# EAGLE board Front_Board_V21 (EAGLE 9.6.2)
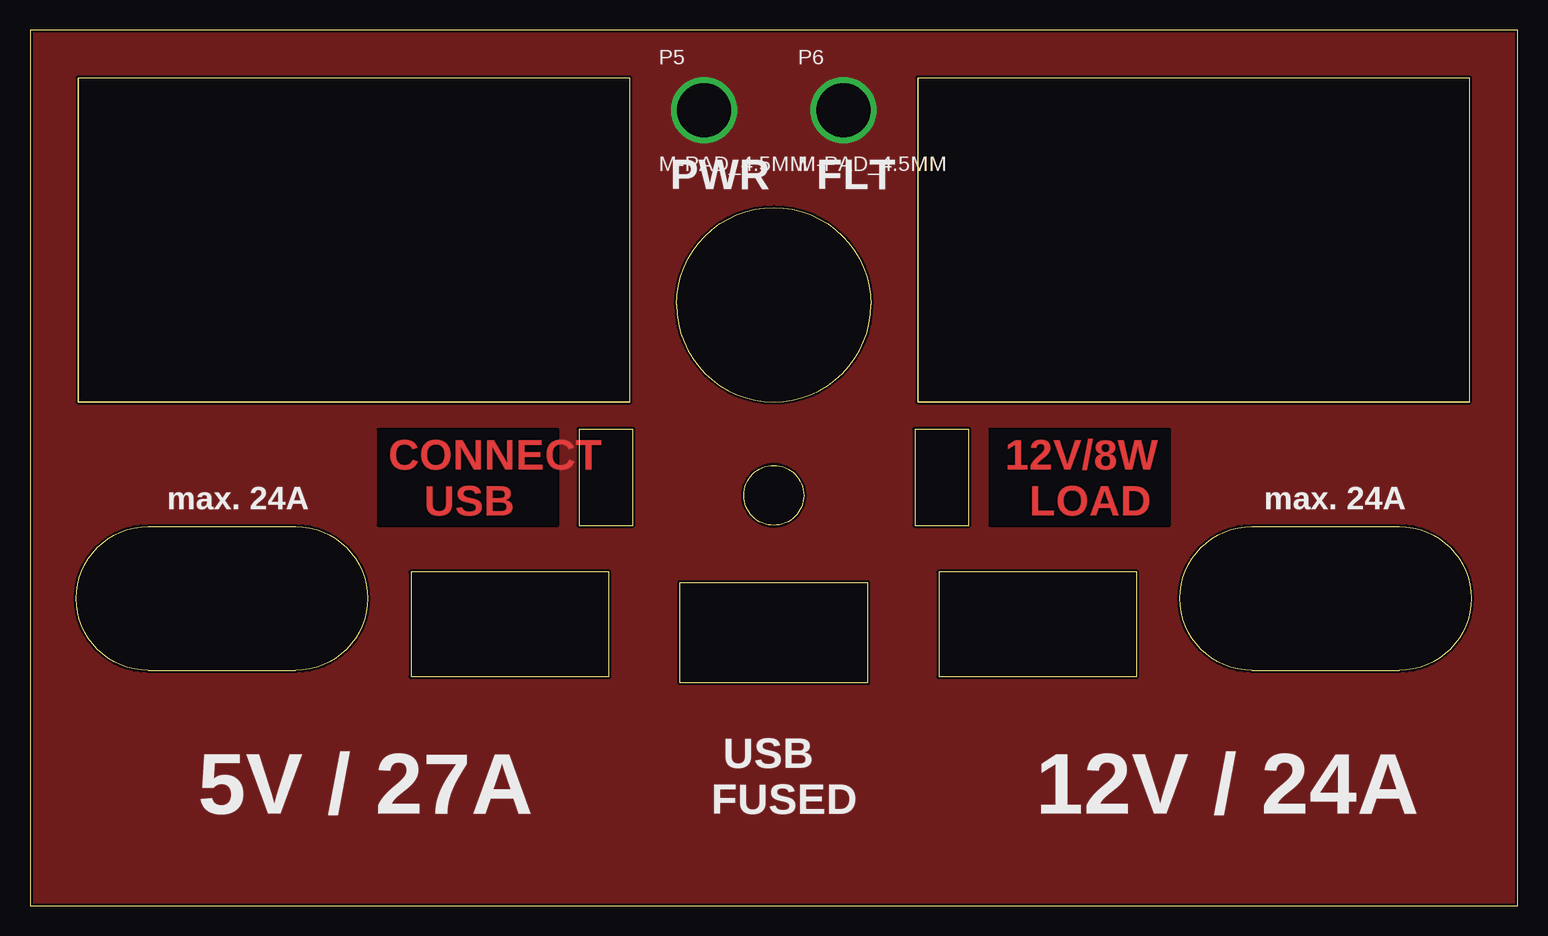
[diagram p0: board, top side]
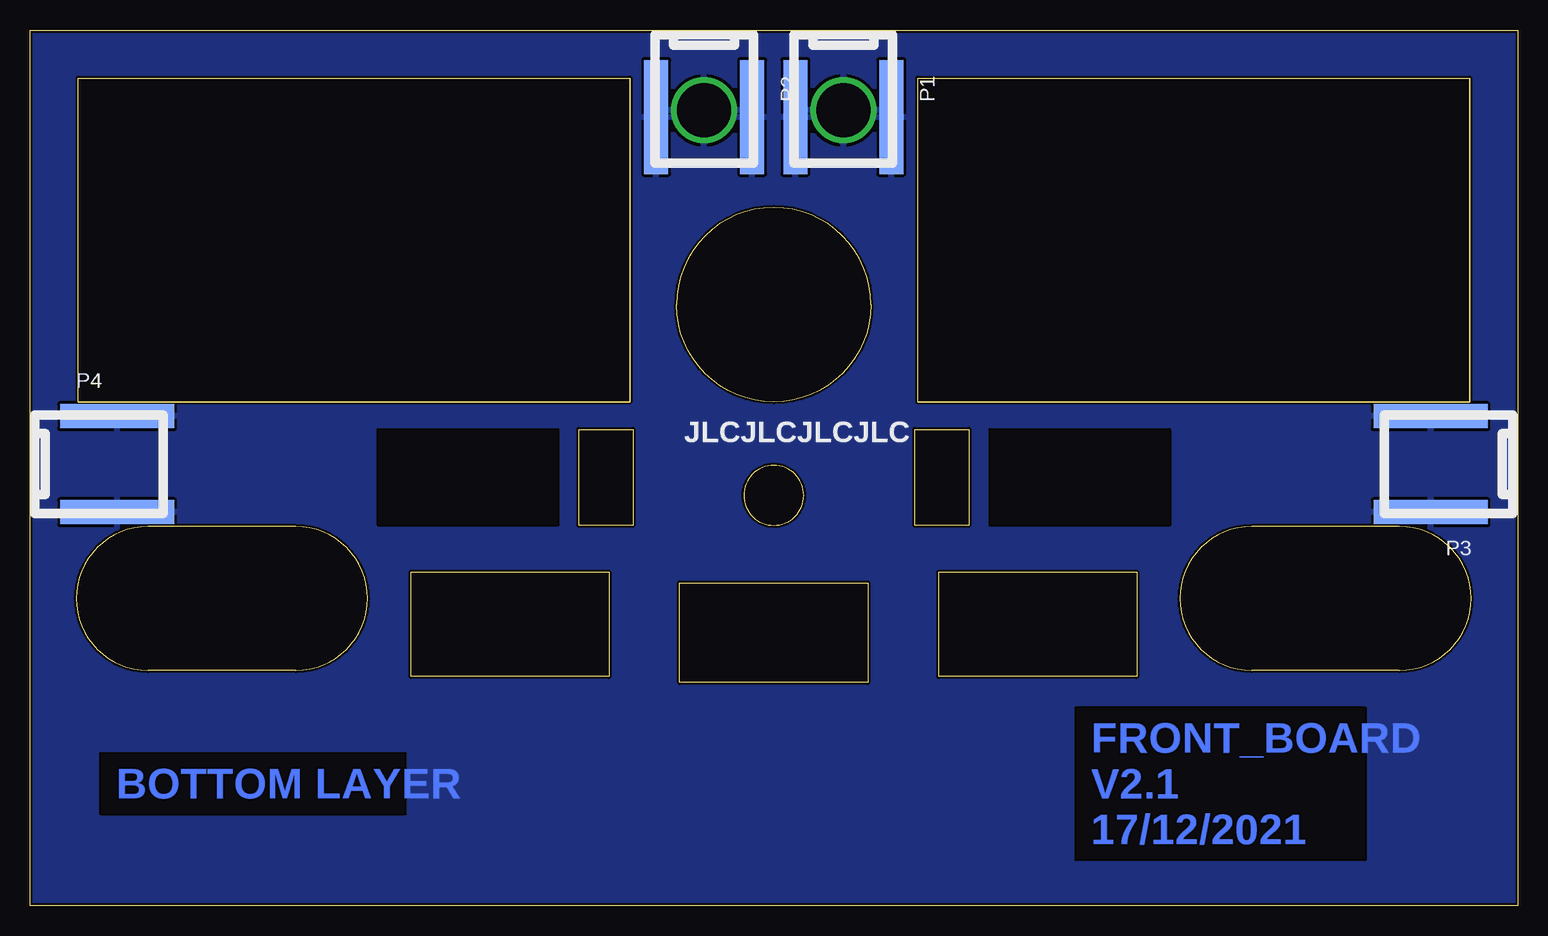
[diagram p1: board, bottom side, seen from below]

Size 124 x 73 mm. Coordinates in mm from the lower left corner, seen from the top.
Outline: 0,0 124,0 124,73 0,73 0,0
Outline: 53.9,50.1 arc-180 70.1,50.1 arc-180 53.9,50.1
Outline: 4,42 50,42 50,69 4,69 4,42
Outline: 74,42 120,42 120,69 74,69 74,42
Outline: 9.85,19.6 arc-180 9.85,31.6 22.15,31.6 arc-180 22.15,19.6 9.85,19.6
Outline: 101.85,19.6 arc-180 101.85,31.6 114.15,31.6 arc-180 114.15,19.6 101.85,19.6
Outline: 31.75,19.1 48.25,19.1 48.25,27.8 31.75,27.8 31.75,19.1
Outline: 75.75,19.1 92.25,19.1 92.25,27.8 75.75,27.8 75.75,19.1
Outline: 54.15,18.6 69.85,18.6 69.85,26.9 54.15,26.9 54.15,18.6
Outline: 59.5,34.2 arc-180 64.5,34.2 arc-180 59.5,34.2
Outline: 45.75,31.7 50.25,31.7 50.25,39.7 45.75,39.7 45.75,31.7
Outline: 73.75,31.7 78.25,31.7 78.25,39.7 73.75,39.7 73.75,31.7
Copper layers (1*16): Top 0.035mm / dielectric 1.5mm / Bottom 0.035mm
Design rules "JLCPCB_2alyer": minimum track width 5mil, minimum drill 0.2mm, track to track 5mil, track to pad 0.2mm, pad to pad 0.2mm, via to via 0.2mm, smd to smd 5mil, copper to edge 0.2mm, drill to drill 0.5mm, minimum pad ring 0.13mm, minimum via ring 0.13mm, stop-mask expansion 0.05mm, vias tented up to drill 0mil, thermal gap 10mil
tRestrict: 8 lines
bRestrict: 16 lines
Milling: 40 lines

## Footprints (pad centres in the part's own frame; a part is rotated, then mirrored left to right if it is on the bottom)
KEYSTONE_7761_PCB-SCREW_M3_SMD = smd 9.5 x 2: P$1 7.25,-4; P$2 7.25,4
M-PAD_4.5MM = drill 4.5 pad 5.1: P$1 0,0

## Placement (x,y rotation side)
P1  KEYSTONE_7761_PCB-SCREW_M3_SMD  [KEYSTONE_7761_PCB-SCREW_M3_SMD]  56.2,73 270 bottom
P2  KEYSTONE_7761_PCB-SCREW_M3_SMD  [KEYSTONE_7761_PCB-SCREW_M3_SMD]  67.8,73 270 bottom
P3  KEYSTONE_7761_PCB-SCREW_M3_SMD  [KEYSTONE_7761_PCB-SCREW_M3_SMD]  0,36.8 180 bottom
P4  KEYSTONE_7761_PCB-SCREW_M3_SMD  [KEYSTONE_7761_PCB-SCREW_M3_SMD]  124,36.8 0 bottom
P5  M-PAD_4.5MM  [M-PAD_4.5MM]  56.2,66.3 0 top
P6  M-PAD_4.5MM  [M-PAD_4.5MM]  67.8,66.3 0 top

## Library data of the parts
P1-P6 = Antec-Hood

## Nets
GND: P1.P$1 P1.P$2 P2.P$1 P2.P$2 P3.P$1 P3.P$2 P4.P$1 P4.P$2 P5.P$1 P6.P$1

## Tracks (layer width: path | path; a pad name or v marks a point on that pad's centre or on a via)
GND
  pour Bottom: -3.81,77.47 -3.81,-5.08 -2.54,-6.35 125.73,-6.35 128.27,-3.81 128.27,77.47 127,78.74 -2.54,78.74
  pour Top (no thermals): -2.54,76.2 -2.54,-5.08 125.73,-5.08 127,-3.81 128.27,-2.54 128.27,77.47 0,77.47 -1.27,77.47

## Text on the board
Top: CONNECT / USB | 12V/8W / LOAD
Bottom: BOTTOM LAYER | FRONT_BOARD / V2.1 / 17/12/2021
tPlace: PWR | FLT | max. 24A | max. 24A | 5V / 27A | USB / FUSED | 12V / 24A
bPlace: JLCJLCJLCJLC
